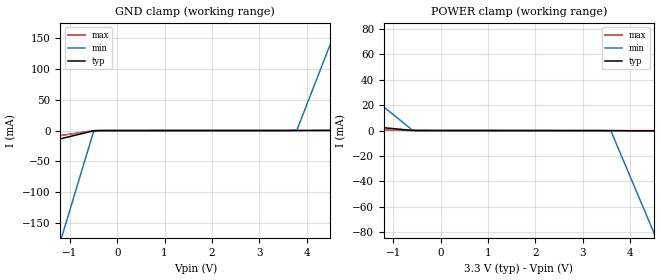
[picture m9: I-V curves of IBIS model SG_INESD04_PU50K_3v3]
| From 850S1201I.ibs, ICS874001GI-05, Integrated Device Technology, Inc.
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[Model] SG_INESD04_PU50K_3v3
Model_type   Input
Polarity   Non-Inverting
Vinl = 0.80V
Vinh = 2.2V
|   typ   min   max
C_comp   2pF   1.5pF   2.5pF
|   typ   min   max
[Voltage range]  3.3V   3.15V   3.45V
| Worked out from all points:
|   GND clamp passes 1 mA (typ) near -0.53 V on its own axis
|   POWER clamp passes 1 mA (typ) near -0.87 V on its own axis
[GND_clamp]
|Voltage   I(typ)   I(min)   I(max)
-3.3V     -52.32mA   -711.5mA   -31.62mA
-1.2V     -13.41mA   -179.2mA   -8.071mA
-1.1V     -11.55mA   -153.8mA   -6.95mA
-500mV    -433.8uA   -1.71mA    -222.1uA
-300mV    -72.6uA    -79.63uA   -71.42uA
3.6V      5.971uA    25.79uA    2.555uA
3.8V      12.83uA    1.398mA    6.341uA
4.6V      337.5uA    158.9mA    21.57uA
4.7V      378uA      178.5mA    23.48uA
6.6V      1.149mA    552.5mA    59.65uA
[POWER_clamp]
|Voltage   I(typ)   I(min)   I(max)
-3.3V     9.672mA    81.68mA    1.945mA
-600mV    53.4uA     339.2uA    15.55uA
3.4V      -67.68uA   -73.38uA   -64.41uA
3.6V      -72.6uA    -756.6uA   -68.21uA
4.5V      -313.7uA   -80.25mA   -85.33uA
4.6V      -340.5uA   -89.08mA   -87.23uA
6.6V      -876.2uA   -265.7mA   -125.3uA
